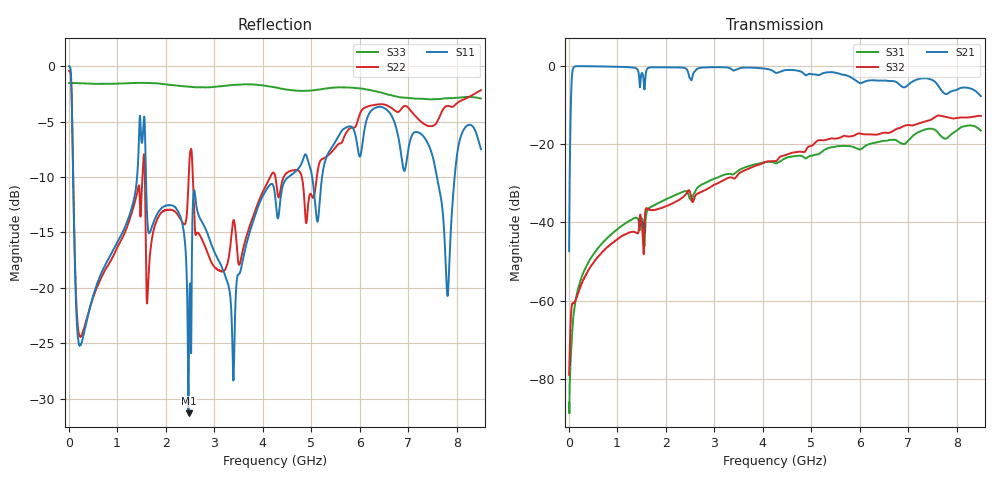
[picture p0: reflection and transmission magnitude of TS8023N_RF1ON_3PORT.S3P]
!Agilent Technologies,E5071C,MY46522130,B.12.04
!Date: Thu Jul 17 20:31:46 2025
!Data & Calibration Information:
!Freq	S11:SOLT3(ON)	S13:SOLT3(ON)	S14:SOLT3(ON)
!	S31:SOLT3(ON)	S33:SOLT3(ON)	S34:SOLT3(ON)
!	S41:SOLT3(ON)	S43:SOLT3(ON)	S44:SOLT3(ON)
!PortZ  Port1:50+j0  Port3:50+j0  Port4:50+j0
!Above PortZ is port z conversion or system Z0 setting when saving the data.
!When reading, reference impedance value at option line is always used.
# Hz S dB R 50
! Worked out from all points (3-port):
!   1601 points, 10 MHz to 8.5 GHz, reference 50 ohm
!   strongest paths, dB at 10 MHz, 2.132 GHz, 4.255 GHz, 6.378 GHz, 8.5 GHz:
!     S21: -47.4, -0.5, -1.8, -3.8, -7.8
!     S32: -79.0, -35.2, -24.4, -17.6, -12.9
!     S31: -86.1, -33.4, -24.9, -19.5, -16.6
!   lowest |S11| = -31.3 dB at 2.472 GHz (marker M1), VSWR 1.06, Z = 50.8 - j2.62 ohm
!   |S11| at or under -10 dB: 92.9 MHz to 1.411 GHz (1.319 GHz wide, 175 % of centre); 1.594 GHz to 4.535 GHz (2.94 GHz wide, 95.9 % of centre); 7.594 GHz to 7.959 GHz (364.5 MHz wide, 4.69 % of centre)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
1e7  0.00 163.0  -47.41 -110.8  -86.97 82.3
     -47.39 -110.6  -0.42 162.0  -77.51 -109.4
     -86.07 69.6  -78.98 -100.3  -1.52 179.8
6.836875e7  -3.80 42.9  -2.70 128.9  -69.50 -89.3
            -2.70 128.8  -3.84 35.5  -60.82 135.2
            -68.87 -88.8  -61.03 134.9  -1.52 179.1
1.267375e8  -17.58 -18.9  -0.25 60.5  -61.45 166.8
            -0.25 60.5  -16.93 -36.5  -60.27 100.2
            -61.43 167.1  -60.47 100.3  -1.53 178.3
4.238875e8  -22.10 -66.4  -0.19 9.1  -49.87 112.4
            -0.19 9.1  -22.01 -86.2  -51.94 94.8
            -49.85 112.2  -51.87 95.4  -1.57 174.4
1.522281e9  -6.65 -106.7  -2.04 -28.4  -39.26 89.6
            -2.05 -28.4  -9.97 -146.2  -42.58 81.6
            -39.29 89.5  -42.63 81.2  -1.50 159.0
2.4721e9  -31.33 -71.5  -2.16 -54.7  -33.03 81.8
          -2.16 -54.7  -10.29 -122.1  -31.88 88.5
          -33.03 82.0  -31.85 88.8  -1.85 147.0
4.255e9  -11.62 155.3  -1.75 -83.8  -25.02 65.4
         -1.76 -83.8  -9.85 -167.2  -24.51 73.0
         -24.93 65.7  -24.42 73.2  -1.91 123.3
6.494238e9  -3.75 142.1  -3.85 -122.9  -19.27 30.0
            -3.82 -123.2  -3.45 154.3  -17.12 21.8
            -19.22 29.5  -17.15 21.9  -2.44 92.8
7.810188e9  -20.73 128.4  -7.31 -145.2  -18.57 12.1
            -7.21 -145.0  -3.59 111.8  -13.22 -13.0
            -18.47 11.1  -13.19 -13.6  -2.90 60.5
8.5e9  -7.48 100.3  -7.79 -159.0  -16.65 -10.4
       -7.82 -158.7  -2.16 104.3  -12.96 -22.8
       -16.57 -9.8  -12.86 -22.6  -2.92 56.9
